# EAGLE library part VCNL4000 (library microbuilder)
VCNL4000 - I²C Proximity and Light Sensor Supply: 2.5-3.6V Proximity: up to 200mm Luminosity: 0.25 to 16,000 lux (16-bit values) Digikey: 751-1505-1-ND
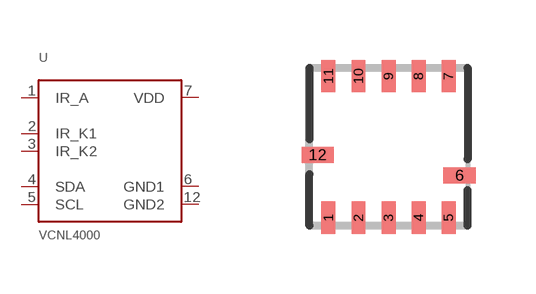
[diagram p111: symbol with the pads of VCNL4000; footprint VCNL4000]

Designator prefix U

## VCNL4000  [VCNL4000]
1  IR_A
2  IR_K1
3  IR_K2
4  SDA
5  SCL
6  GND1
7  VDD
12  GND2

## Footprint VCNL4000 (pad centres in mm)
Source: http://www.vishay.com/docs/83798/vcnl4000.pdf
smd 0.35 x 0.805: 1 -1.5,-1.772; 2 -0.75,-1.772; 3 0,-1.772; 4 0.75,-1.772; 5 1.5,-1.772; 7 1.5,1.772; 8 0.75,1.772; 9 0,1.772; 10 -0.75,1.772; 11 -1.5,1.772
smd 0.805 x 0.4: 6 1.772,-0.715; 12 -1.772,-0.2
